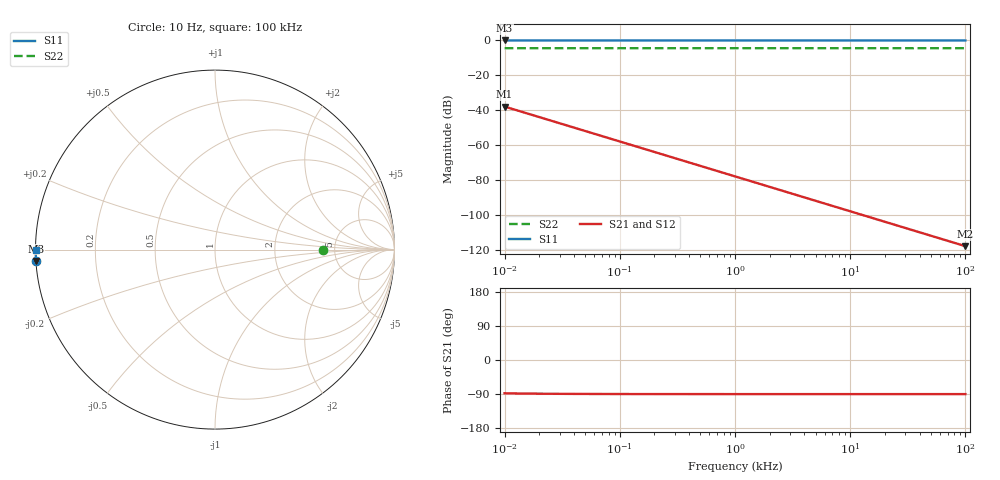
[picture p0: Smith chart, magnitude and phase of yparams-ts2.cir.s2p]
[Version] 2.0
# Hz Y RI R 50
[Number of Ports] 2
[Two-Port Data Order] 12_21
[Reference] 50 50
!  Freq  ReY11  ImY11  ReY12  ImY12  ReY21  ImY21  ReY22  ImY22
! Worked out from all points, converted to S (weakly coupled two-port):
!   41 points, 10 Hz to 100 kHz, reference 50 ohm
!   highest |S21| = -37.91 dB at 10 Hz (marker M1); lowest = -117.9 dB at 100 kHz (marker M2)
!   lowest |S11| = 0.0 dB at 10 Hz (marker M3)
!   |S11| at or under -10 dB: nowhere
!   |S22| runs from -4.4 to -4.4 dB; largest |S21 - S12| = 3.4e-17
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[Number of Frequencies] 22
[Network Data]
10  0.0129 0.6281  -0.005 6.28e-05  -0.005 6.28e-05  0.005 6.53e-09
12.58925  0.0175 0.7907  -0.005 7.91e-05  -0.005 7.91e-05  0.005 8.22e-09
15.84893  0.0248 0.9952  -0.005 9.95e-05  -0.005 9.95e-05  0.005 1.03e-08
19.95262  0.0364 1.253  -0.005 0.000125  -0.005 0.000125  0.005 1.3e-08
25.11886  0.0548 1.576  -0.00499 0.000158  -0.00499 0.000158  0.005 1.64e-08
31.62278  0.0838 1.983  -0.00499 0.000198  -0.00499 0.000198  0.005 2.06e-08
39.81072  0.1298 2.495  -0.00499 0.000249  -0.00499 0.000249  0.005 2.59e-08
50.11872  0.2025 3.136  -0.00498 0.000314  -0.00498 0.000314  0.005 3.26e-08
63.09573  0.3173 3.939  -0.00497 0.000394  -0.00497 0.000394  0.005 4.1e-08
79.43282  0.4981 4.941  -0.00495 0.000494  -0.00495 0.000494  0.005 5.14e-08
100  0.7821 6.184  -0.00492 0.000618  -0.00492 0.000618  0.005 6.43e-08
125.8925  1.225 7.715  -0.00488 0.000772  -0.00488 0.000772  0.005 8.03e-08
158.4893  1.912 9.576  -0.00481 0.000958  -0.00481 0.000958  0.005 9.97e-08
251.1886  4.534 14.35  -0.00455 0.00144  -0.00455 0.00144  0.005 1.5e-07
316.2278  6.822 17.16  -0.00432 0.00172  -0.00432 0.00172  0.005 1.79e-07
501.1872  14.2 22.54  -0.00358 0.00225  -0.00358 0.00225  0.005 2.38e-07
794.3282  24.95 25  -0.0025 0.0025  -0.0025 0.0025  0.005 2.7e-07
1258.925  35.72 22.58  -0.00143 0.00226  -0.00143 0.00226  0.005 2.57e-07
1584.893  39.93 20.05  -0.00101 0.002  -0.00101 0.002  0.005 2.4e-07
5011.872  48.77 7.744  -0.000123 0.000774  -0.000123 0.000774  0.005 2.02e-07
25118.86  49.95 1.582  -5.01e-06 0.000158  -5.01e-06 0.000158  0.005 6.39e-07
100000  50 0.3979  -3.09e-07 3.98e-05  -3.09e-07 3.98e-05  0.005 2.49e-06
[End]
